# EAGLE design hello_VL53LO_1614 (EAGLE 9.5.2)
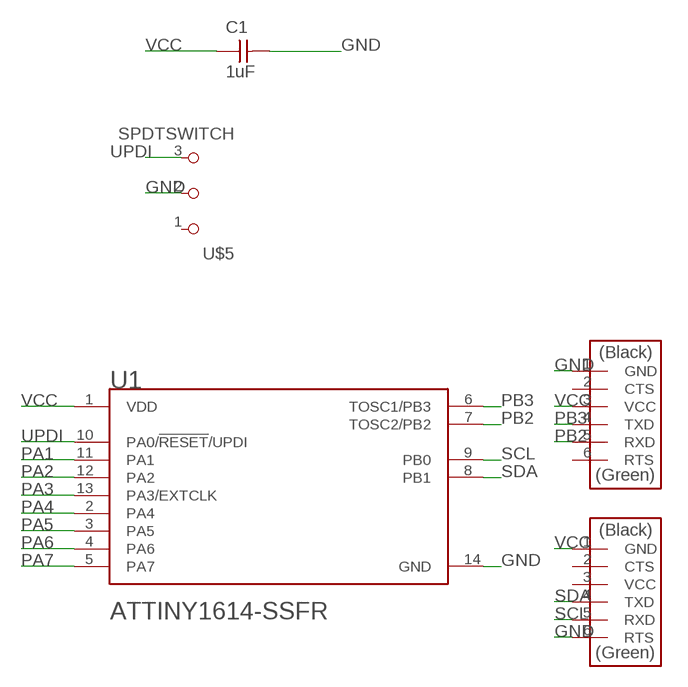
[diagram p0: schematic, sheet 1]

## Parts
C1  1uF  CAP_UNPOLARIZEDFAB  [C1206FAB]
U1  MICROCHIP_ATTINY1614-SSFRMICROCHIP_ATTINY1614-SSFR_0_1  [MICROCHIP_ATTINY1614]
U$1  CONN_06_FTDI-SMD-HEADER  [1X06SMD]
U$2  CONN_06_FTDI-SMD-HEADER  [1X06SMD]
U$5  SPDTSWITCH  [SPDTSWITCH]

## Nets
GND: C1.2 U1.14(GND) U$1.6(RTS) U$2.1(GND) U$5.2
PA1: U1.11(PA1)
PA2: U1.12(PA2)
PA3: U1.13(PA3/EXTCLK)
PA4: U1.2(PA4)
PA5: U1.3(PA5)
PA6: U1.4(PA6)
PA7: U1.5(PA7)
PB2: U1.7(TOSC2/PB2) U$2.5(RXD)
PB3: U1.6(TOSC1/PB3) U$2.4(TXD)
SCL: U1.9(PB0) U$1.5(RXD)
SDA: U1.8(PB1) U$1.4(TXD)
UPDI: U1.10(PA0/!RESET!/UPDI) U$5.3
VCC [New Class]: C1.1 U1.1(VDD) U$1.1(GND) U$2.3(VCC)
Unconnected: U$1.2(CTS) U$1.3(VCC) U$2.2(CTS) U$2.6(RTS) U$5.1

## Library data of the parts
C1 = fab:CAP_UNPOLARIZED
U1 = Microchip - ATTINY1614-SSFR:MICROCHIP_ATTINY1614-SSFR: IC MCU 8BIT 16KB FLASH 14SOIC; AUTOMOTIVE: No; CENTROID_NOT_SPECIFIED: No; CORE_ARCHITECTURE: AVR; DATASHEET: http://ww1.microchip.com/downloads/en/DeviceDoc/ATtiny1614-DataSheet-DS40001995B.pdf; DATA_BUS_WIDTH: 8bits; DEVICE_CLASS_L1: Integrated Circuits (ICs); DEVICE_CLASS_L2: Embedded Processors and Controllers; DEVICE_CLASS_L3: Microcontrollers; DIGIKEY_DESCRIPTION: IC MCU 8BIT 16KB FLASH 14SOIC; DIGIKEY_PART_NUMBER: ATTINY1614-SSFRCT-ND; FOOTPRINT_PARAMETERS_1: {"fp_type":"SOIC_narrow","params":{"N":{"nom":14,"long name":"Number of leads","min":null,"max":null,"short name":"N","type":"count"},"A":{"nom":false,"long name":"Height","min":false,"max":1750000,"short name":"A","type":"measurement"},"A1":{"nom":false,"long name":"Package clearance","min":100000,"max":250000,"short name":"A1","type":"measurement"},"A2":{"nom":false,"long name":"Package height","min":1250000,"max":false,"short name":"A2","type":"measurement"},"D":{"nom":8650000,"long name":"Package length","min":8550000,"max":8750000,"short name":"D","type":"measurement"},"E":{"nom":6000000,"long name":"Width w/ leads","min":5800000,"max":6200000,"short name":"E","type":"measurement"},"E1":{"nom":3900000,"long name":"Package width","min":3800000,"max":4000000,"short name":"E1","type":"measurement"},"B":{"nom":false,"long name":"Lead width","min":310000,"max":510000,"short name":"B","type":"measurement"},"C":{"nom":false,"long name":"Lead thickness","min":100000,"max":250000,"short name":"C","type":"measurement"},"e":{"nom":1270000,"long name":"Lead pitch","min":null,"max":null,"short name":"e","type":"measurement"},"L":{"nom":false,"long name":"Lead foot length","min":400000,"max":1270000,"short name":"L","type":"measurement"},"PHI":{"nom":false,"long name":"Lead foot angle","min":0,"max":8000000,"short name":"PHI","type":"measurement"},"HT":{"default":"No","long name":"Thermal pad","type":"multichoiceparent","short name":"HT","children":[]},"offset x":{"nom":0,"long name":"X Center offset","min":null,"max":null,"short name":"offset x","type":"measurement"},"offset y":{"nom":0,"long name":"Y Center offset","min":null,"max":null,"short name":"offset y","type":"measurement"},"LS":{"default":"Rounded rectangle","long name":"Land shape","type":"multichoice","short name":"LS"},"LS1":{"default":"Rectangle","long name":"Land shape (Pin 1)","type":"multichoice","short name":"LS1"},"solder toe":{"nom":550000,"long name":"Solder fillet (toe)","min":null,"max":null,"short name":"solder toe","type":"fixedmeasurement"},"solder heel":{"nom":450000,"long name":"Solder fillet (heel)","min":null,"max":null,"short name":"solder heel","type":"fixedmeasurement"},"solder side":{"nom":50000,"long name":"Solder fillet (side)","min":null,"max":null,"short name":"solder side","type":"fixedmeasurement"},"courtyard":{"nom":500000,"long name":"Courtyard","min":null,"max":null,"short name":"courtyard","type":"fixedmeasurement"},"SF":{"default":"A","long name":"Packing level","type":"multichoiceparent","short name":"SF","help":"http://support.upverter.com/customer/portal/articles/978783-what-is-a-footprint-packing-level","children":["solder toe","solder heel","solder side","courtyard"]}}}; FOOTPRINT_PARAMETERS_2: {"fp_type":"SOIC_narrow","params":{"N":{"nom":14,"long name":"Number of leads","min":null,"max":null,"short name":"N","type":"count"},"A":{"nom":false,"long name":"Height","min":false,"max":1750000,"short name":"A","type":"measurement"},"A1":{"nom":false,"long name":"Package clearance","min":100000,"max":250000,"short name":"A1","type":"measurement"},"A2":{"nom":false,"long name":"Package height","min":1250000,"max":false,"short name":"A2","type":"measurement"},"D":{"nom":8650000,"long name":"Package length","min":8550000,"max":8750000,"short name":"D","type":"measurement"},"E":{"nom":6000000,"long name":"Width w/ leads","min":5800000,"max":6200000,"short name":"E","type":"measurement"},"E1":{"nom":3900000,"long name":"Package width","min":3800000,"max":4000000,"short name":"E1","type":"measurement"},"B":{"nom":false,"long name":"Lead width","min":310000,"max":510000,"short name":"B","type":"measurement"},"C":{"nom":false,"long name":"Lead thickness","min":100000,"max":250000,"short name":"C","type":"measurement"},"e":{"nom":1270000,"long name":"Lead pitch","min":null,"max":null,"short name":"e","type":"measurement"},"L":{"nom":false,"long name":"Lead foot length","min":400000,"max":1270000,"short name":"L","type":"measurement"},"PHI":{"nom":false,"long name":"Lead foot angle","min":0,"max":8000000,"short name":"PHI","type":"measurement"},"HT":{"default":"No","long name":"Thermal pad","type":"multichoiceparent","short name":"HT","children":[]},"offset x":{"nom":0,"long name":"X Center offset","min":null,"max":null,"short name":"offset x","type":"measurement"},"offset y":{"nom":0,"long name":"Y Center offset","min":null,"max":null,"short name":"offset y","type":"measurement"},"LS":{"default":"Rounded rectangle","long name":"Land shape","type":"multichoice","short name":"LS"},"LS1":{"default":"Rectangle","long name":"Land shape (Pin 1)","type":"multichoice","short name":"LS1"},"solder toe":{"nom":350000,"long name":"Solder fillet (toe)","min":null,"max":null,"short name":"solder toe","type":"fixedmeasurement"},"solder heel":{"nom":350000,"long name":"Solder fillet (heel)","min":null,"max":null,"short name":"solder heel","type":"fixedmeasurement"},"solder side":{"nom":30000,"long name":"Solder fillet (side)","min":null,"max":null,"short name":"solder side","type":"fixedmeasurement"},"courtyard":{"nom":250000,"long name":"Courtyard","min":null,"max":null,"short name":"courtyard","type":"fixedmeasurement"},"SF":{"default":"B","long name":"Packing level","type":"multichoiceparent","short name":"SF","help":"http://support.upverter.com/customer/portal/articles/978783-what-is-a-footprint-packing-level","children":["solder toe","solder heel","solder side","courtyard"]}}}; FOOTPRINT_PARAMETERS_3: {"fp_type":"SOIC_narrow","params":{"N":{"nom":14,"long name":"Number of leads","min":null,"max":null,"short name":"N","type":"count"},"A":{"nom":false,"long name":"Height","min":false,"max":1750000,"short name":"A","type":"measurement"},"A1":{"nom":false,"long name":"Package clearance","min":100000,"max":250000,"short name":"A1","type":"measurement"},"A2":{"nom":false,"long name":"Package height","min":1250000,"max":false,"short name":"A2","type":"measurement"},"D":{"nom":8650000,"long name":"Package length","min":8550000,"max":8750000,"short name":"D","type":"measurement"},"E":{"nom":6000000,"long name":"Width w/ leads","min":5800000,"max":6200000,"short name":"E","type":"measurement"},"E1":{"nom":3900000,"long name":"Package width","min":3800000,"max":4000000,"short name":"E1","type":"measurement"},"B":{"nom":false,"long name":"Lead width","min":310000,"max":510000,"short name":"B","type":"measurement"},"C":{"nom":false,"long name":"Lead thickness","min":100000,"max":250000,"short name":"C","type":"measurement"},"e":{"nom":1270000,"long name":"Lead pitch","min":null,"max":null,"short name":"e","type":"measurement"},"L":{"nom":false,"long name":"Lead foot length","min":400000,"max":1270000,"short name":"L","type":"measurement"},"PHI":{"nom":false,"long name":"Lead foot angle","min":0,"max":8000000,"short name":"PHI","type":"measurement"},"HT":{"default":"No","long name":"Thermal pad","type":"multichoiceparent","short name":"HT","children":[]},"offset x":{"nom":0,"long name":"X Center offset","min":null,"max":null,"short name":"offset x","type":"measurement"},"offset y":{"nom":0,"long name":"Y Center offset","min":null,"max":null,"short name":"offset y","type":"measurement"},"LS":{"default":"Rounded rectangle","long name":"Land shape","type":"multichoice","short name":"LS"},"LS1":{"default":"Rectangle","long name":"Land shape (Pin 1)","type":"multichoice","short name":"LS1"},"solder toe":{"nom":150000,"long name":"Solder fillet (toe)","min":null,"max":null,"short name":"solder toe","type":"fixedmeasurement"},"solder heel":{"nom":250000,"long name":"Solder fillet (heel)","min":null,"max":null,"short name":"solder heel","type":"fixedmeasurement"},"solder side":{"nom":10000,"long name":"Solder fillet (side)","min":null,"max":null,"short name":"solder side","type":"fixedmeasurement"},"courtyard":{"nom":100000,"long name":"Courtyard","min":null,"max":null,"short name":"courtyard","type":"fixedmeasurement"},"SF":{"default":"C","long name":"Packing level","type":"multichoiceparent","short name":"SF","help":"http://support.upverter.com/customer/portal/articles/978783-what-is-a-footprint-packing-level","children":["solder toe","solder heel","solder side","courtyard"]}}}; FOOTPRINT_VARIANT_NAME_0: Recommended_Land_Pattern; FOOTPRINT_VARIANT_NAME_1: IPC_A; FOOTPRINT_VARIANT_NAME_2: IPC_B; FOOTPRINT_VARIANT_NAME_3: IPC_C; FREQUENCY: 16MHz; HEIGHT: 1.75mm; INTERFACE: I2C,SPI,UART,USART,2-Wire,LIN,IrDA; IPC_LAND_PATTERN_NAME: SOIC127P600X175-14; LEAD_FREE: Yes; MAX_SUPPLY_VOLTAGE: 5.5V; MEMORY_SIZE: 16KBytes; MEMORY_TYPE: FLASH; MF: Microchip; MFG_PACKAGE_IDENT: C04-065-D3X; MFG_PACKAGE_IDENT_DATE: 0; MFG_PACKAGE_IDENT_REV: D; MIN_SUPPLY_VOLTAGE: 1.8V; MOUSER_DESCRIPTION: 8-Bit AVR Microcontroller 16Kbyte Flash 2Kbyte SRAM 14-Pin SOIC T/R; MOUSER_PART_NUMBER: 556-ATTINY1614SSFR; MPN: ATTINY1614-SSFR; NOMINAL_SUPPLY_CURRENT: 2.6-10200uA; NUMBER_OF_A/D_CONVERTERS: 2; NUMBER_OF_ADC_CHANNELS: 14; NUMBER_OF_CORES: 1; NUMBER_OF_I/OS: 12; NUMBER_OF_I2C_CHANNELS: 1; NUMBER_OF_PWM_CHANNELS: 1; NUMBER_OF_SPI_CHANNELS: 1; NUMBER_OF_TIMERS/COUNTERS: 5; NUMBER_OF_UART_CHANNELS: 1; PACKAGE: SOIC14; PREFIX: U; RAM_SIZE: 2KBytes; ROHS: Yes; STANDOFF_HEIGHT: 0.1mm; TEMPERATURE_RANGE_HIGH: +125°C; TEMPERATURE_RANGE_LOW: -40°C; VERIFICATION_VERSION: 0.0.0.3
U$1 U$2 = fab:CONN_06_FTDI-SMD-HEADER
U$5 = fab:SPDTSWITCH

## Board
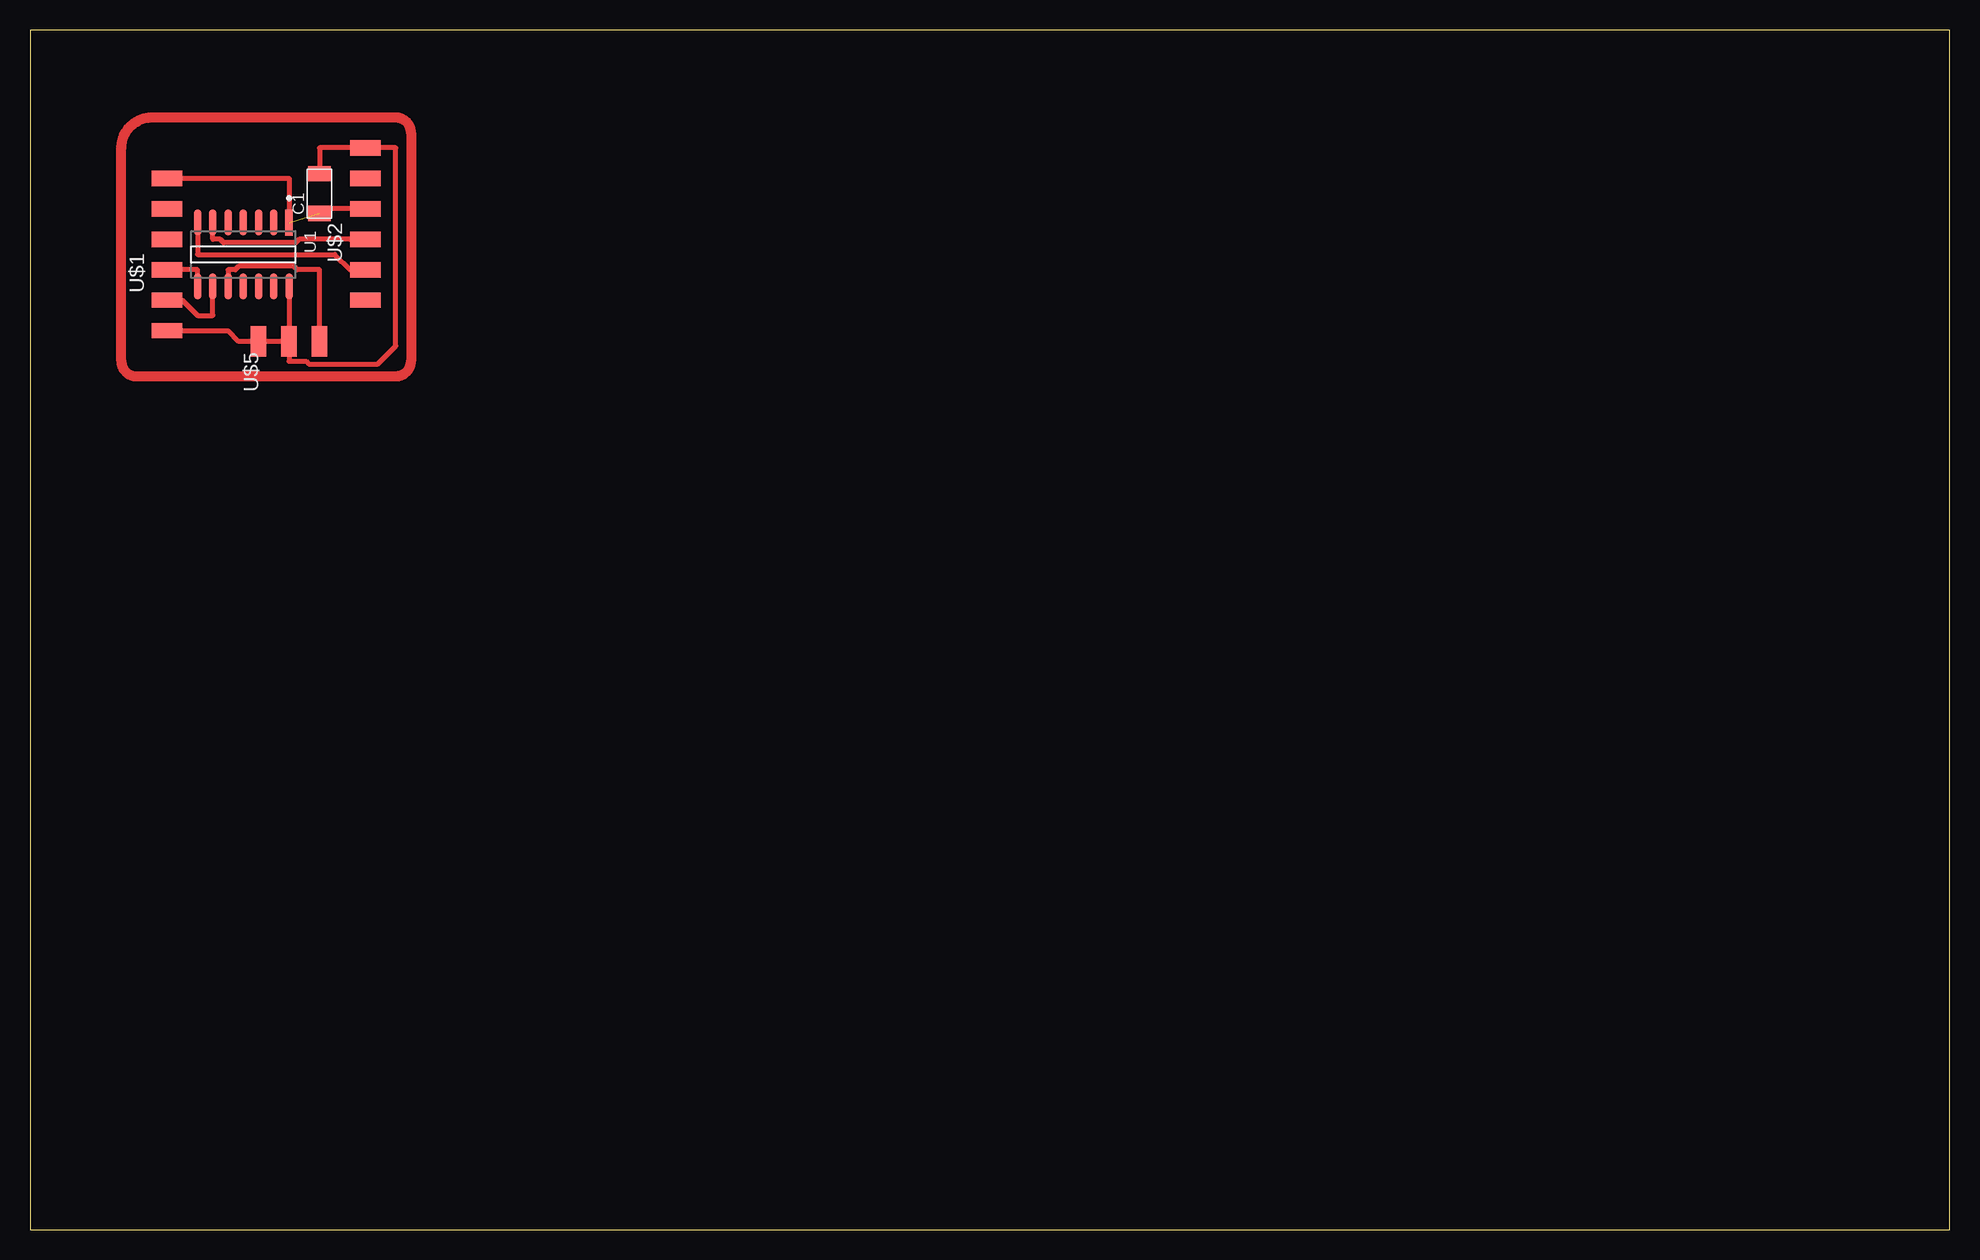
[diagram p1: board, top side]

Size 160 x 100 mm. Coordinates in mm from the lower left corner, seen from the top.
Outline: 0,0 160,0 160,100 0,100 0,0
Copper layers (1*16): Top 0.035mm / dielectric 1.5mm / Bottom 0.035mm
Design rules "default *": minimum track width 16mil, minimum drill 0.35mm, track to track 16mil, track to pad 16mil, pad to pad 16mil, via to via 16mil, smd to smd 16mil, copper to edge 40mil, drill to drill 6mil, minimum pad ring 10mil, minimum via ring 8mil, stop-mask expansion 4mil, vias tented up to drill 0mil, thermal gap 10mil

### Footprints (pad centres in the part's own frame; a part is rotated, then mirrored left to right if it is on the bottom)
C1206FAB = smd 1.27 x 1.905: 1 -1.651,0; 2 1.651,0
MICROCHIP_ATTINY1614 = smd 2.169 x 0.622: 1 -2.67,3.81; 2 -2.67,2.54; 3 -2.67,1.27; 4 -2.67,0; 5 -2.67,-1.27; 6 -2.67,-2.54; 7 -2.67,-3.81; 8 2.67,-3.81; 9 2.67,-2.54; 10 2.67,-1.27; 11 2.67,0; 12 2.67,1.27; 13 2.67,2.54; 14 2.67,3.81
1X06SMD = smd 2.54 x 1.27: 1 0,6.35; 2 0,3.81; 3 0,1.27; 4 0,-1.27; 5 0,-3.81; 6 0,-6.35
SPDTSWITCH = smd 2.54 x 1.27: 1 0.38,2.54; 2 0.38,0; 3 0.38,-2.54

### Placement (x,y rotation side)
C1  24.13,86.36 90 top
U1  17.78,81.28 270 top
U$1  11.43,81.28 0 top
U$2  27.94,83.82 0 top
U$5  21.59,73.66 90 top

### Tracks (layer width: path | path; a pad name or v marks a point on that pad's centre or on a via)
GND
  Top 0.406: U$1.6 16.51,74.93 17.4,74.04 U$5.2 | U$5.2 21.59,73.66 | C1.2 24.13,90.17 U$2.1 30.48,90.17 30.48,73.66 28.98,72.16 23.24,72.16 23.01,72.39 21.59,72.39 U$5.2 | U$5.2 21.97,73.66 | U1.14 U$5.2
N$2
  Top 0.813: 7.62,90.17 arc-90 10.16,92.71 30.48,92.71 arc-90 31.75,91.44 31.75,72.39 arc-90 30.48,71.12 8.89,71.12 arc-90 7.62,72.39 7.62,90.17
PB2
  Top 0.406: U1.7 13.97,81.28 25.4,81.28 26.67,80.01 U$2.5
PB3
  Top 0.406: 26.67,82.55 U$2.4 22.45,82.55 22.15,82.26 16.13,82.26 15.83,82.55 15.24,82.55 U1.6
SCL
  Top 0.406: 11.84,77.88 U$1.5 12.7,77.47 13.97,76.2 15.24,76.2 U1.9
SDA
  Top 0.406: U1.8 13.97,80.01 U$1.4
UPDI
  Top 0.406: 24.13,73.82 U$5.3 24.13,80.01 22.27,80.01 21.97,80.3 17.4,80.3 17.1,80.01 16.51,80.01 U1.10
VCC  (1 unrouted)
  Top 0.406: U$2.3 24.51,85.09 C1.1 | U$1.1 21.59,87.63 U1.1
